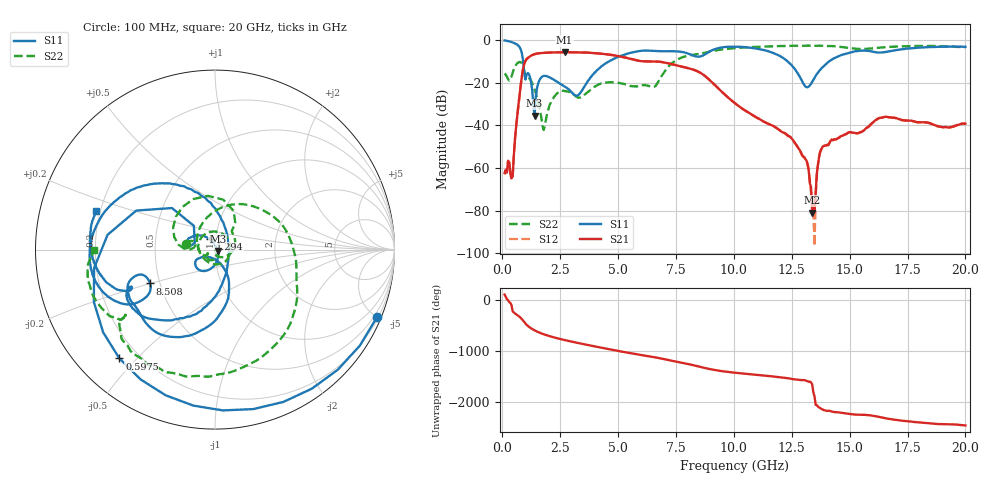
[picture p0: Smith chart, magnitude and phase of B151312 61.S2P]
!  2-Port S-parameters saved by WinCal
! VAR MeasName=S-Parameters (CALIBRATED_DATA) read from VNA (N5244A)
! VAR MeasDate=12/8/2015 5:48:34 PM
! VAR NAME=B151312 61
! VAR FILENAME=B151312 61.S2P
! VAR DATE=12/8/2015 5:48:34 PM
! VAR PHYS_PORTS=1,2
# Hz S DB R 50
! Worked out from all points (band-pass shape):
!   401 points, 100 MHz to 20 GHz, reference 50 ohm
!   highest |S21| = -5.72 dB at 2.687 GHz (marker M1); lowest = -80.9 dB at 13.38 GHz (marker M2)
!   |S21| within 3 dB of the highest: 1.074 GHz to 5.501 GHz (4.428 GHz wide, 135 % of centre)
!   lowest |S11| = -35.5 dB at 1.393 GHz (marker M3), VSWR 1.03, Z = 51.6 - j0.723 ohm
!   |S11| at or under -10 dB: 900.1 MHz to 4.61 GHz (3.71 GHz wide, 135 % of centre); 12.32 GHz to 14.12 GHz (1.8 GHz wide, 13.6 % of centre)
!   |S22| runs from -42.2 to -2.6 dB; largest |S21 - S12| = 0.0018
!   S11 on the Smith chart (normalised r, x): 100 MHz: 0.29, -4.99; 597.5 MHz: 0.13, -0.45; 1.294 GHz: 0.94, +0.11; 8.508 GHz: 0.44, -0.20; 20 GHz: 0.18, +0.15
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1e8  -0.20 -22.6  -62.31 110.6  -63.04 110.1  -15.67 168.6
3.985e8  -0.94 -87.2  -64.73 -97.3  -65.60 -109.8  -17.13 179.9
5.975e8  -1.86 -131.3  -40.63 82.0  -40.65 82.8  -11.57 152.1
8.96e8  -9.54 136.0  -13.64 -42.3  -13.64 -42.3  -12.40 64.3
1.294e9  -23.78 114.7  -7.04 151.0  -7.05 151.0  -20.26 -6.4
1.3935e9  -35.45 -24.5  -6.62 125.3  -6.62 125.3  -23.08 -34.3
1.7915e9  -16.84 -127.9  -6.02 47.4  -6.02 47.4  -42.22 -70.0
2.1895e9  -18.38 -151.1  -5.81 -8.8  -5.81 -8.8  -27.53 -70.2
2.687e9  -21.78 -149.2  -5.72 -66.1  -5.73 -66.1  -23.93 -128.0
3.43325e9  -23.82 -78.3  -5.82 -140.1  -5.82 -140.0  -26.56 -149.3
4.7765e9  -9.02 -84.7  -7.10 98.9  -7.08 98.8  -19.84 107.4
5.672e9  -5.66 -110.9  -9.18 24.2  -9.17 24.2  -21.68 1.2
6.7665e9  -5.22 -140.1  -10.16 -62.0  -10.15 -62.1  -18.98 153.8
7.41325e9  -5.24 -150.4  -11.56 -122.0  -11.55 -122.2  -10.18 53.3
8.50775e9  -7.79 -152.4  -15.09 129.7  -15.09 129.4  -6.48 -17.0
1.005e10  -3.10 -177.1  -29.62 9.3  -29.60 8.7  -3.79 -64.3
1.25375e10  -12.31 92.9  -46.72 -116.8  -46.80 -117.0  -2.68 -111.5
1.31345e10  -22.07 12.5  -56.49 -150.6  -56.56 -148.0  -2.61 -119.9
1.338325e10  -19.60 -47.2  -80.91 139.4  -76.81 147.5  -2.68 -122.9
1.388075e10  -12.22 -87.1  -49.66 -5.8  -49.54 -5.8  -2.67 -129.8
1.67165e10  -5.32 -154.9  -36.29 178.3  -36.18 177.9  -3.20 -147.5
2e10  -3.17 162.1  -39.26 49.9  -39.30 49.4  -3.40 -179.6
